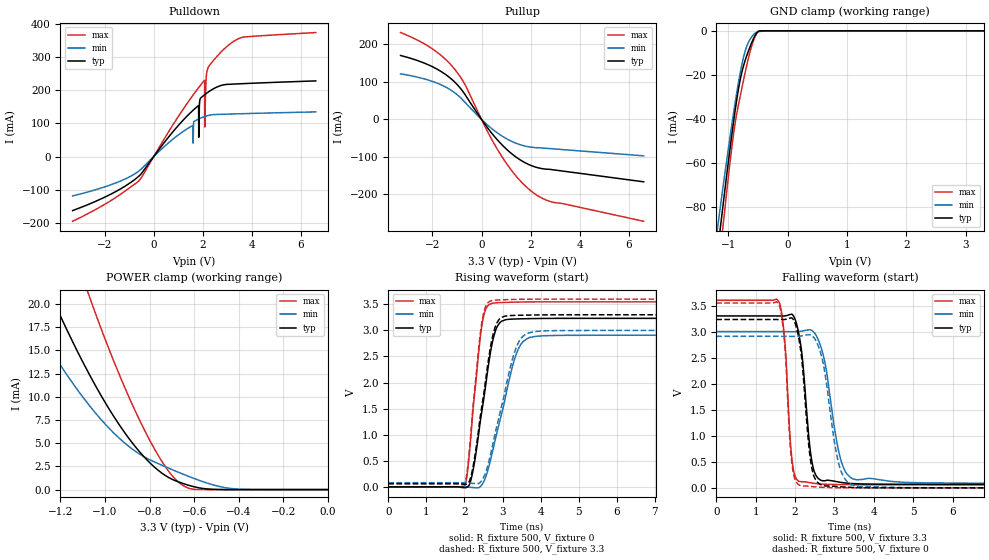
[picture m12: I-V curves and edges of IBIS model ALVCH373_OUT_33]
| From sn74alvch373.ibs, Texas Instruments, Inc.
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[Model]   ALVCH373_OUT_33
Model_type  3-state
Enable   Active-Low
Vref =   0
Rref =   500
Cref =   50p
Vmeas =   1.5
| variable   typ   min   max
C_comp   6.47pF   5.63pF   7.59pF
| C_pullup   8.37pF   6.58pF   9.47pF
| C_pulldown   15.41pF   1.42pF   38.08pF
| C_tri-state   6.47pF   5.63pF   7.59pF
[Temperature Range]   40   100   -40
| Ambient temperature   25   85   -40
[Voltage range]   3.3   3   3.6
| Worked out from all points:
|   slope of the pulldown table from 0 to 0.495 V, typ, clamps not added: 10.2 ohm
|   slope of the pullup table from 0 to 0.495 V, typ, clamps not added: 11.5 ohm
|   GND clamp passes 1 mA (typ) near -0.52 V on its own axis
|   POWER clamp passes 1 mA (typ) near -0.69 V on its own axis
|   rising waveform, R_fixture 500, V_fixture 0: 20-80 % time 383ps typ, 560ps min, 273ps max; typ from 0 V to 3.23 V
|   falling waveform, R_fixture 500, V_fixture 3.3: 20-80 % time 227ps typ, 364ps min, 163ps max; typ from 3.3 V to 0.064 V
|   rising waveform, R_fixture 500, V_fixture 3.3: 20-80 % time 378ps typ, 551ps min, 271ps max; typ from 0.064 V to 3.3 V
|   falling waveform, R_fixture 500, V_fixture 0: 20-80 % time 221ps typ, 342ps min, 161ps max; typ from 3.23 V to 0 V
[GND Clamp]
| ALVCH373_OUT_33
|   Voltage   I(typ)   I(min)   I(max)
-3.3V     -639.1mA   -566.5mA   -715mA
-1.18V    -100.5mA   -89.65mA   -112.8mA
-1.125V   -87.85mA   -78.5mA    -98.43mA
-1.1V     -82.17mA   -73.5mA    -91.99mA
-1.075V   -76.54mA   -68.54mA   -85.62mA
-900mV    -39.46mA   -35.65mA   -44.99mA
-795mV    -21.86mA   -18.76mA   -29.33mA
-725mV    -14.35mA   -10.23mA   -20.24mA
-665mV    -9.566mA   -5.551mA   -13.05mA
-565mV    -3.023mA   -1.514mA   -3.748mA
-485mV    -120.2uA   -421uA     -114.9uA
3.3V      139.3pA    2.386uA    18.29pA
[POWER Clamp]
| ALVCH373_OUT_33
|   Voltage   I(typ)   I(min)   I(max)
-3.3V     184.2mA    138.4mA    249.4mA
-1.385V   29.11mA    20.85mA    44.74mA
-1.235V   20.55mA    14.71mA    32.69mA
-1.1V     13.76mA    9.984mA    22.84mA
-1.065V   12.17mA    8.905mA    20.46mA
-975mV    8.428mA    6.446mA    14.71mA
-875mV    4.956mA    4.322mA    9.027mA
-765mV    2.151mA    2.842mA    3.833mA
-670mV    829.8uA    1.861mA    798.1uA
-600mV    303.5uA    1.195mA    26.53uA
-440mV    2.059uA    132.1uA    46.49nA
-48.03fV  139.3pA    693.1pA    20.85pA
[Pulldown]
| ALVCH373_OUT_33
|   Voltage   I(typ)   I(min)   I(max)
-3.3V     -162.1mA   -118mA     -194.3mA
-590mV    -57.85mA   -42.71mA   -71.5mA
1.815V    152.9mA    112.5mA    205.9mA
1.83V     153.5mA    113.1mA    207.4mA
1.835V    58.23mA    113.3mA    207.9mA
1.875V    167.7mA    114.6mA    211.7mA
2.075V    186.2mA    120.5mA    229.6mA
2.08V     186.5mA    120.7mA    229mA
2.085V    186.7mA    120.8mA    88.86mA
2.19V     192.5mA    123.1mA    262.2mA
3.1V      217.6mA    128mA      338.4mA
6.6V      227.7mA    134.5mA    373mA
[Pullup]
| ALVCH373_OUT_33
|   Voltage   I(typ)   I(min)   I(max)
-3.3V     170.6mA    121.7mA    231.7mA
-2.03V    141.5mA    102.1mA    189.4mA
-1.535V   123.1mA    88.81mA    164.3mA
-1.115V   101mA      72.26mA    135.6mA
-680mV    66.96mA    46.06mA    93.77mA
200mV     -18.44mA   -12.39mA   -26.59mA
790mV     -64.77mA   -42.41mA   -95.13mA
1.42V     -101mA     -63.79mA   -152.1mA
2.05V     -123.6mA   -74.17mA   -192.5mA
2.45V     -130.9mA   -75.99mA   -209.4mA
2.85V     -133.6mA   -78.01mA   -219.7mA
6.6V      -166.2mA   -96.97mA   -271.5mA
[Ramp]
| ALVCH373_OUT_33
| variable   typ   min   max
dV/dt_r   1.95/3.87E-10   1.76/5.64E-10   2.14/2.76E-10
dV/dt_f   1.96/2.38E-10   1.77/3.78E-10   2.14/1.66E-10
R_load = 500
[Rising Waveform]
| ALVCH373_OUT_33
R_fixture =   500
C_fixture =   0
L_fixture =   0
V_fixture =   0
V_fixture_min = 0
V_fixture_max = 0
|   Time   V(typ)   V(min)   V(max)
0s        63.31pV    2.907nV    51.87pV
1.995ns   -12.72mV   234.1uV    8.849mV
2.08ns    2.175mV    -3.611mV   292.7mV
2.19ns    192.2mV    -10.6mV    1.161V
2.47ns    1.511V     53.88mV    3.147V
2.585ns   2.094V     247.7mV    3.445V
2.81ns    2.982V     908.9mV    3.529V
3.39ns    3.221V     2.598V     3.543V
3.9ns     3.228V     2.889V     3.547V
40ns      3.232V     2.909V     3.548V
[Falling Waveform]
| ALVCH373_OUT_33
R_fixture =   500
C_fixture =   0
L_fixture =   0
V_fixture =   3.3
V_fixture_min = 3
V_fixture_max = 3.6
|   Time   V(typ)   V(min)   V(max)
0s        3.3V       3V         3.6V
1.605ns   3.299V     3V         3.545V
1.74ns    3.3V       2.999V     2.81V
1.96ns    3.299V     2.997V     341.1mV
2.155ns   2.683V     3.007V     117.2mV
2.38ns    758.5mV    3.034V     100.1mV
2.545ns   222.6mV    2.912V     81.04mV
3.155ns   106.3mV    556mV      62.51mV
3.57ns    78.76mV    154.5mV    60.17mV
40ns      63.74mV    79.96mV    56.07mV
[Rising Waveform]
| ALVCH373_OUT_33
R_fixture =   500
C_fixture =   0
L_fixture =   0
V_fixture =   3.3
V_fixture_min = 3
V_fixture_max = 3.6
|   Time   V(typ)   V(min)   V(max)
0s        63.74mV    79.9mV     56.07mV
1.995ns   50.88mV    79.74mV    65.09mV
2.08ns    66.37mV    75.82mV    350.9mV
2.19ns    259.6mV    68.95mV    1.23V
2.46ns    1.56V      126.4mV    3.167V
2.58ns    2.174V     326.4mV    3.494V
2.79ns    3.024V     968.4mV    3.579V
3.39ns    3.289V     2.721V     3.596V
4.005ns   3.298V     2.987V     3.599V
40ns      3.3V       3V         3.6V
[Falling Waveform]
| ALVCH373_OUT_33
R_fixture =   500
C_fixture =   0
L_fixture =   0
V_fixture =   0
V_fixture_min = 0
V_fixture_max = 0
|   Time   V(typ)   V(min)   V(max)
0s        3.232V     2.909V     3.548V
1.6ns     3.23V      2.908V     3.498V
1.74ns    3.232V     2.908V     2.726V
1.92ns    3.261V     2.906V     461.3mV
2.16ns    2.539V     2.916V     39.25mV
2.485ns   211.3mV    2.877V     21.41mV
2.715ns   45.72mV    2.387V     9.488mV
3.135ns   22.17mV    389.4mV    2.846mV
3.62ns    5.034mV    27.07mV    932.3uV
40ns      638nV      4.838uV    251.3nV
